TYPE ST_Channel :
STRUCT
	(* Acceleration, mean of acc, std of acc, ... ; velocity, mean of ... *)
	AccRMS				: LREAL;
	AccMeanRMS			: LREAL;
	AccStdRMS			: LREAL;
	AccMeanPlusStdRms	: LREAL;
	AccMeanMinusStdRms	: LREAL;
	
	VelRMS				: LREAL;
	VelMeanRMS			: LREAL;
	VelStdRMS			: LREAL;
	VelMeanPlusStdRms	: LREAL;
	VelMeanMinusStdRms	: LREAL;
	
	DispRMS				: LREAL;
	DispMeanRMS			: LREAL;
	DispStdRMS			: LREAL;
	DispMeanPlusStdRms	: LREAL;
	DispMeanMinusStdRms	: LREAL;
END_STRUCT
END_TYPE
